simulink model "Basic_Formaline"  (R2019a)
settings: Solver=VariableStepAuto  StartTime=0.0  StopTime=10.0  RelTol=1e-3
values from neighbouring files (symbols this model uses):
  Cv = u(2)    [valve.m]
  delta_p = u(3)    [valve.m]
  valve_type = 3    [Valve_script.m]
  x_MeOHsp = u(1)    [Bias_calc.m]
undefined symbols (not defined in the file or in its folder): air_fan, F_MeOHsp, mixerMeOH_O2, par_valve_actuator, valve, valve0, valve_actuator
libraries: simulink x2

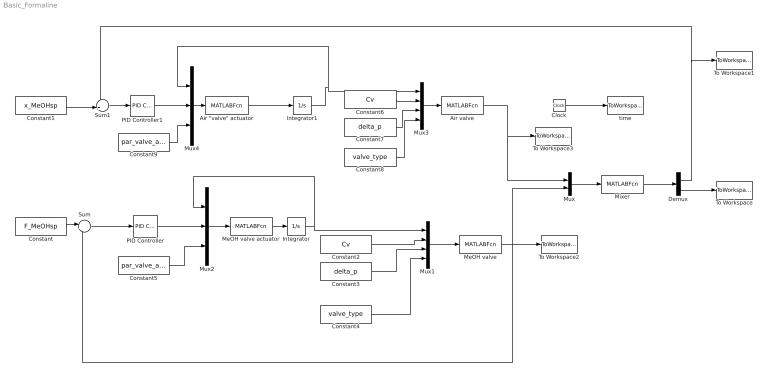
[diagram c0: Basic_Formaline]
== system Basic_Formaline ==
  "Air \"valve\" actuator" : MATLABFcn  MATLABFcn=air_fan(u)  OutputDimensions=1
  Air valve : MATLABFcn  MATLABFcn=valve(u)  OutputDimensions=1
  Clock : Clock
  Constant : Constant  Value=F_MeOHsp
  Constant1 : Constant  Value=x_MeOHsp
  Constant2 : Constant  Value=Cv
  Constant3 : Constant  Value=delta_p
  Constant4 : Constant  Value=valve_type
  Constant5 : Constant  Value=par_valve_actuator
  Constant6 : Constant  Value=Cv
  Constant7 : Constant  Value=delta_p
  Constant8 : Constant  Value=valve_type
  Constant9 : Constant  Value=par_valve_actuator
  Demux : Demux  Outputs=2
  Integrator : Integrator  InitialCondition=valve0
  Integrator1 : Integrator  InitialCondition=valve0
  MeOH valve : MATLABFcn  MATLABFcn=valve(u)  OutputDimensions=1
  MeOH valve actuator : MATLABFcn  MATLABFcn=valve_actuator(u(1:2),u(3),u(4:6))  OutputDimensions=1
  Mixer : MATLABFcn  MATLABFcn=mixerMeOH_O2(u)  OutputDimensions=2
  Mux : Mux  Inputs=2
  Mux1 : Mux
  Mux2 : Mux  Inputs=3
  Mux3 : Mux
  Mux4 : Mux  Inputs=3
  PID Controller : simulink/Continuous/PID Controller  Controller=PI  Form=Parallel  TimeDomain=Continuous-time  SampleTime=-1  IntegratorMethod=Forward Euler  FilterMethod=Forward Euler  ControllerParametersSource=internal  P=1  I=1  D=0  UseFilter=on  N=100  TunerSelectOption=Transfer Function Based (PID Tuner App)  InitialConditionSource=internal  InitialConditionForIntegrator=0  InitialConditionForFilter=0  DifferentiatorICPrevScaledInput=0  ExternalReset=none  TrackingMode=off  Kt=1  LimitOutput=off  UpperSaturationLimit=inf  LowerSaturationLimit=-inf  LinearizeAsGain=on  AntiWindupMode=none  Kb=1  POutMin=[]  POutMax=[]  IOutMin=[]  IOutMax=[]  DOutMin=[]  DOutMax=[]  NOutMin=[]  NOutMax=[]  SumOutMin=[]  SumOutMax=[]  SaturationOutMin=[]  SaturationOutMax=[]  PParamMin=[]  PParamMax=[]  IParamMin=[]  IParamMax=[]  DParamMin=[]  DParamMax=[]  NParamMin=[]  NParamMax=[]  KbParamMin=[]  KbParamMax=[]  KtParamMin=[]  KtParamMax=[]  KbOutMin=[]  KbOutMax=[]  KtOutMin=[]  KtOutMax=[]  IntegratorOutMin=[]  IntegratorOutMax=[]  FilterOutMin=[]  FilterOutMax=[]  SumI1OutMin=[]  SumI1OutMax=[]  SumI2OutMin=[]  SumI2OutMax=[]  SumI3OutMin=[]  SumI3OutMax=[]  SumI4OutMin=[]  SumI4OutMax=[]  SumDOutMin=[]  SumDOutMax=[]  DifferentiatorOutMin=[]  DifferentiatorOutMax=[]  FilterDiffOutCoefMin=[]  FilterDiffOutCoefMax=[]  ReciprocalOutMin=[]  ReciprocalOutMax=[]  SumDenOutMin=[]  SumDenOutMax=[]  SumNumOutMin=[]  SumNumOutMax=[]  DivideOutMin=[]  DivideOutMax=[]  IntegratorContinuousStateAttributes=''  IntegratorStateMustResolveToSignalObject=off  IntegratorRTWStateStorageClass=Auto  FilterContinuousStateAttributes=''  FilterStateMustResolveToSignalObject=off  FilterRTWStateStorageClass=Auto  ParallelPVariant=InternalParameters  IdealPVariant=Disabled  IVariant=InternalParameters  DVariant=Disabled  IntegratorVariant=Continuous  SatVariant=Disabled  AWVariant=Passthrough  PCopyVariant=Disabled  TRVariant=Disabled  FdbkBlocksVariant=Forward  IdealPFdbkVariant=Disabled  SatFdbkVariant=Disabled  DerivativeFilterVariant=Disabled  NVariant=Disabled  NCopyVariant=Disabled_SignalSpec  FilterICVariant=Disabled  IntegratorICVariant=InternalICs  ExternalResetVariant=Disabled  TRSumVariant=Passthrough  SumFdbkVariant=Disabled  SumVariant=Sum_PI
  PID Controller1 : simulink/Continuous/PID Controller  Controller=PI  Form=Parallel  TimeDomain=Continuous-time  SampleTime=-1  IntegratorMethod=Forward Euler  FilterMethod=Forward Euler  ControllerParametersSource=internal  P=1  I=1  D=0  UseFilter=on  N=100  TunerSelectOption=Transfer Function Based (PID Tuner App)  InitialConditionSource=internal  InitialConditionForIntegrator=0  InitialConditionForFilter=0  DifferentiatorICPrevScaledInput=0  ExternalReset=none  TrackingMode=off  Kt=1  LimitOutput=off  UpperSaturationLimit=inf  LowerSaturationLimit=-inf  LinearizeAsGain=on  AntiWindupMode=none  Kb=1  POutMin=[]  POutMax=[]  IOutMin=[]  IOutMax=[]  DOutMin=[]  DOutMax=[]  NOutMin=[]  NOutMax=[]  SumOutMin=[]  SumOutMax=[]  SaturationOutMin=[]  SaturationOutMax=[]  PParamMin=[]  PParamMax=[]  IParamMin=[]  IParamMax=[]  DParamMin=[]  DParamMax=[]  NParamMin=[]  NParamMax=[]  KbParamMin=[]  KbParamMax=[]  KtParamMin=[]  KtParamMax=[]  KbOutMin=[]  KbOutMax=[]  KtOutMin=[]  KtOutMax=[]  IntegratorOutMin=[]  IntegratorOutMax=[]  FilterOutMin=[]  FilterOutMax=[]  SumI1OutMin=[]  SumI1OutMax=[]  SumI2OutMin=[]  SumI2OutMax=[]  SumI3OutMin=[]  SumI3OutMax=[]  SumI4OutMin=[]  SumI4OutMax=[]  SumDOutMin=[]  SumDOutMax=[]  DifferentiatorOutMin=[]  DifferentiatorOutMax=[]  FilterDiffOutCoefMin=[]  FilterDiffOutCoefMax=[]  ReciprocalOutMin=[]  ReciprocalOutMax=[]  SumDenOutMin=[]  SumDenOutMax=[]  SumNumOutMin=[]  SumNumOutMax=[]  DivideOutMin=[]  DivideOutMax=[]  IntegratorContinuousStateAttributes=''  IntegratorStateMustResolveToSignalObject=off  IntegratorRTWStateStorageClass=Auto  FilterContinuousStateAttributes=''  FilterStateMustResolveToSignalObject=off  FilterRTWStateStorageClass=Auto  ParallelPVariant=InternalParameters  IdealPVariant=Disabled  IVariant=InternalParameters  DVariant=Disabled  IntegratorVariant=Continuous  SatVariant=Disabled  AWVariant=Passthrough  PCopyVariant=Disabled  TRVariant=Disabled  FdbkBlocksVariant=Forward  IdealPFdbkVariant=Disabled  SatFdbkVariant=Disabled  DerivativeFilterVariant=Disabled  NVariant=Disabled  NCopyVariant=Disabled_SignalSpec  FilterICVariant=Disabled  IntegratorICVariant=InternalICs  ExternalResetVariant=Disabled  TRSumVariant=Passthrough  SumFdbkVariant=Disabled  SumVariant=Sum_PI
  Sum : Sum  Inputs=|+-
  Sum1 : Sum  Inputs=-+|
  To Workspace : ToWorkspace  VariableName=F_tot  SampleTime=-1
  To Workspace1 : ToWorkspace  VariableName=x_MeOH  SampleTime=-1
  To Workspace2 : ToWorkspace  VariableName=F_MeOH  SampleTime=-1
  To Workspace3 : ToWorkspace  VariableName=F_air  SampleTime=-1
  time : ToWorkspace  VariableName=t  SampleTime=-1
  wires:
  Mux/1 -> Mixer/1
  MeOH valve/1 -> Mux/2, To Workspace2/1, Sum/2
  Sum/1 -> PID Controller/1
  Constant/1 -> Sum/1
  Constant1/1 -> Sum1/2
  Sum1/1 -> PID Controller1/1
  Mixer/1 -> Demux/1
  Demux/1 -> To Workspace1/1, Sum1/1
  Clock/1 -> time/1
  Demux/2 -> To Workspace/1
  Air valve/1 -> To Workspace3/1, Mux/1
  Mux1/1 -> MeOH valve/1
  Constant2/1 -> Mux1/2
  Constant3/1 -> Mux1/3
  Constant4/1 -> Mux1/4
  MeOH valve actuator/1 -> Integrator/1
  Mux2/1 -> MeOH valve actuator/1
  Integrator/1 -> Mux2/1, Mux1/1
  Constant5/1 -> Mux2/3
  PID Controller/1 -> Mux2/2
  Mux3/1 -> Air valve/1
  Constant6/1 -> Mux3/2
  Constant7/1 -> Mux3/3
  Constant8/1 -> Mux3/4
  Integrator1/1 -> Mux4/1, Mux3/1
  Mux4/1 -> "Air \"valve\" actuator"/1
  Constant9/1 -> Mux4/3
  PID Controller1/1 -> Mux4/2
  "Air \"valve\" actuator"/1 -> Integrator1/1
